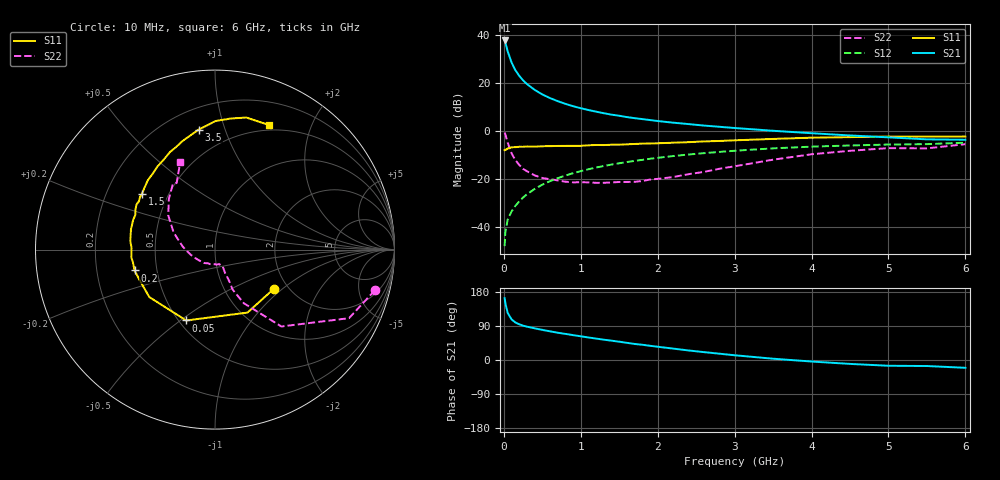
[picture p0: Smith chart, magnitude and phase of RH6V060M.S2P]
! SIEMENS Small Signal Semiconductors
! BFR106
! Si NPN RF Bipolar Junction Transistor in SOT23
! VCE = 6 V  IC = 60 mA
! Common Emitter S-Parameters:  August  1996
# GHz  S  MA  R  50
!  f  S11  S21  S12  S22
! GHz  MAG  ANG  MAG  ANG  MAG  ANG  MAG  ANG
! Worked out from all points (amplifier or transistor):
!   36 points, 10 MHz to 6 GHz, reference 50 ohm
!   highest |S21| = 37.7 dB at 10 MHz (marker M1)
!   |S21| within 3 dB of that: start of sweep to 37.31 MHz
!   unconditionally stable (mu >= 1): 237.8 MHz to 2.294 GHz
!   at 250 MHz: K = 1.01, MAG = 23.8 dB, |S12| = -27.9 dB
!   at 1.4 GHz: K = 1.06, MAG = 9.0 dB, |S12| = -14.1 dB
!   at 6 GHz: K = 0.98, MSG = 0.6 dB, |S12| = -5.0 dB
!   S11 on the Smith chart (normalised r, x): 10 MHz: 1.69, -0.87; 50 MHz: 0.54, -0.53; 200 MHz: 0.37, -0.11; 1.5 GHz: 0.36, +0.30; 3.5 GHz: 0.33, +0.82; 6 GHz: 0.44, +1.43
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0.01  0.3937 -33.8  76.58 163.1  0.0039 80.5  0.9191 -14.3
0.02  0.3948 -62.7  68.95 149.6  0.0077 69.2  0.8387 -27.1
0.05  0.4263 -112.1  45.45 124.3  0.014 61.6  0.5657 -49.2
0.1  0.4517 -144.2  26.64 107.3  0.0206 61.9  0.3388 -61.8
0.15  0.4541 -158.9  18.34 99.0  0.0271 65.2  0.2434 -66.2
0.2  0.4631 -165.5  14.02 94.3  0.0335 68.4  0.1944 -65.7
0.25  0.4625 -171.1  11.25 90.6  0.0404 69.5  0.1602 -66.1
0.3  0.4681 -174.7  9.438 88.0  0.0472 71.3  0.1429 -66.7
0.4  0.4655 178.7  7.138 83.6  0.0609 72.1  0.1172 -66.0
0.5  0.4746 174.0  5.724 79.5  0.0748 72.3  0.1033 -65.5
0.6  0.477 170.1  4.802 75.7  0.0887 72.0  0.0973 -67.0
0.7  0.4816 166.5  4.146 72.0  0.1024 71.3  0.0921 -70.1
0.9  0.4851 160.2  3.251 65.6  0.1302 68.9  0.0837 -74.3
1.1  0.4967 153.1  2.707 59.4  0.1571 66.6  0.0837 -84.2
1.5  0.5118 142.5  2.054 48.3  0.2095 61.2  0.0852 -104.3
1.7  0.5295 136.5  1.83 42.3  0.2347 58.4  0.0859 -116.9
2.2  0.563 124.8  1.474 30.1  0.296 51.0  0.1079 -146.4
2.8  0.6114 110.7  1.21 16.7  0.3614 42.0  0.1607 -178.5
3.5  0.675 97.7  0.998 3.4  0.4289 31.7  0.2489 157.7
4.5  0.736 83.0  0.797 -10.3  0.4923 17.0  0.3814 132.4
5.5  0.7537 70.7  0.661 -15.9  0.5257 7.3  0.428 119.9
6  0.7566 66.5  0.648 -20.6  0.5634 0.1  0.5245 111.7
